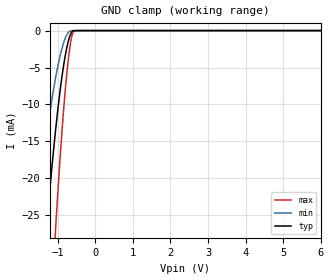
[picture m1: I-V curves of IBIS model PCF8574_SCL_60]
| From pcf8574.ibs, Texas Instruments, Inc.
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[Model]   PCF8574_SCL_60
Model_type  Input
Vinl=1.8
Vinh=4.2
| variable   typ   min   max
C_comp   1.00pF   0.88pF   1.20pF
[Temperature Range]   40   100   -40
| Ambient temperature   25   85   -40
[Voltage range]   6   6   6
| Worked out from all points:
|   GND clamp passes 1 mA (typ) near -0.70 V on its own axis
[GND Clamp]
| PCF8574_SCL_60
|   Voltage   I(typ)   I(min)   I(max)
-6V       -445mA     -305.4mA   -697.7mA
-1.625V   -48.07mA   -27.89mA   -85.05mA
-1.595V   -45.96mA   -26.53mA   -81.6mA
-1.325V   -28.2mA    -15.24mA   -52.18mA
-1.3V     -26.68mA   -14.3mA    -49.62mA
-1.065V   -13.8mA    -6.576mA   -27.43mA
-840mV    -4.575mA   -1.593mA   -10.44mA
-750mV    -2.083mA   -490.5uA   -5.336mA
-675mV    -688uA     -60.7uA    -2.152mA
-615mV    -103.6uA   -20.05uA   -548.3uA
-560mV    -7.89uA    -10.66uA   -15.75uA
6V        519.1pA    651pA      160.9pA
